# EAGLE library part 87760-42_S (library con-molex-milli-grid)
HEADER
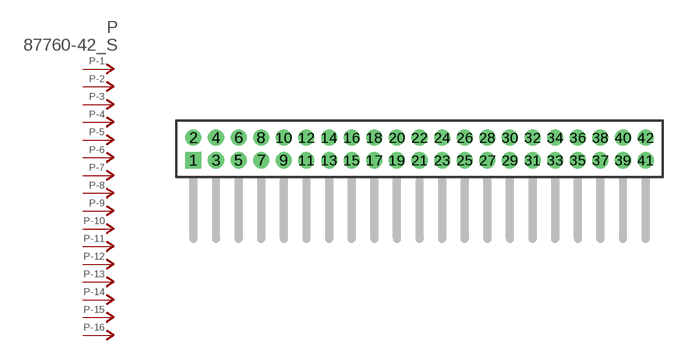
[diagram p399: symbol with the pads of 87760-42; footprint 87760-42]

Designator prefix P; gates -1=P-NV -2=P-N -3=P-N -4=P-N -5=P-N -6=P-N -7=P-N -8=P-N -9=P-N -10=P-N -11=P-N -12=P-N -13=P-N -14=P-N -15=P-N -16=P-N -17=P-N -18=P-N -19=P-N -20=P-N -21=P-N -22=P-N -23=P-N -24=P-N -25=P-N -26=P-N -27=P-N -28=P-N -29=P-N -30=P-N -31=P-N -32=P-N -33=P-N -34=P-N -35=P-N -36=P-N -37=P-N -38=P-N -39=P-N -40=P-N -41=P-N -42=P-N

## 87760-42_S  [87760-42]
1  -1:P  pas
2  -2:P  pas
3  -3:P  pas
4  -4:P  pas
5  -5:P  pas
6  -6:P  pas
7  -7:P  pas
8  -8:P  pas
9  -9:P  pas
10  -10:P  pas
11  -11:P  pas
12  -12:P  pas
13  -13:P  pas
14  -14:P  pas
15  -15:P  pas
16  -16:P  pas
17  -17:P  pas
18  -18:P  pas
19  -19:P  pas
20  -20:P  pas
21  -21:P  pas
22  -22:P  pas
23  -23:P  pas
24  -24:P  pas
25  -25:P  pas
26  -26:P  pas
27  -27:P  pas
28  -28:P  pas
29  -29:P  pas
30  -30:P  pas
31  -31:P  pas
32  -32:P  pas
33  -33:P  pas
34  -34:P  pas
35  -35:P  pas
36  -36:P  pas
37  -37:P  pas
38  -38:P  pas
39  -39:P  pas
40  -40:P  pas
41  -41:P  pas
42  -42:P  pas

## Footprint 87760-42 (pad centres in mm)
HEADER Dual Row, Right Angle
drill 0.914 square: 1 -20,-1
drill 0.914: 2 -20,1; 3 -18,-1; 4 -18,1; 5 -16,-1; 6 -16,1; 7 -14,-1; 8 -14,1; 9 -12,-1; 10 -12,1; 11 -10,-1; 12 -10,1; 13 -8,-1; 14 -8,1; 15 -6,-1; 16 -6,1; 17 -4,-1; 18 -4,1; 19 -2,-1; 20 -2,1; 21 0,-1; 22 0,1; 23 2,-1; 24 2,1; 25 4,-1; 26 4,1; 27 6,-1; 28 6,1; 29 8,-1; 30 8,1; 31 10,-1; 32 10,1; 33 12,-1; 34 12,1; 35 14,-1; 36 14,1; 37 16,-1; 38 16,1; 39 18,-1; 40 18,1; 41 20,-1; 42 20,1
